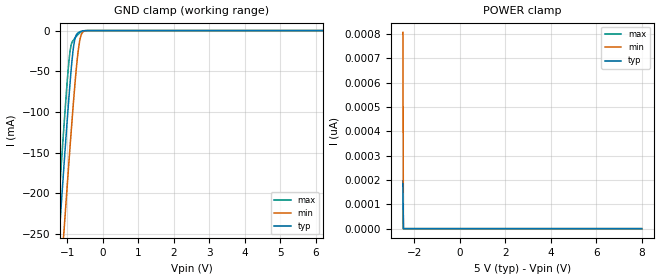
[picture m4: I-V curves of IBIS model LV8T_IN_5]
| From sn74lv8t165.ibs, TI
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[Model]   LV8T_IN_5
Model_type   Input
Vinl = 0.8
Vinh = 2
|   typ   min   max
C_comp   0.94pF   0.94pF   0.94pF
[Voltage Range]   5   4.5   5.5
[Temperature Range]   27   125   -40
[Power Clamp Reference]   5   4.5   5.5
[GND Clamp Reference]   0   0   0
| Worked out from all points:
|   GND clamp passes 1 mA (typ) near -0.62 V on its own axis
[GND Clamp]
|   Voltage   I(typ)   I(min)   I(max)
-2.5V     -1.102A    -1.155A    -1.067A
-1.292V   -294.1mA   -373.9mA   -246.2mA
-1.188V   -226.4mA   -306.9mA   -177.6mA
-1.083V   -160.1mA   -240.9mA   -111mA
-967mV    -90.42mA   -170.1mA   -44.5mA
-914.5mV  -60.98mA   -138.9mA   -23.57mA
-809.5mV  -15.97mA   -79.55mA   -10.72mA
-757mV    -6.46mA    -52.6mA    -7.795mA
-673mV    -2.071mA   -18.84mA   -3.804mA
-599.5mV  -718.5uA   -4.334mA   -1.428mA
-442mV    -12.39uA   -73.18uA   -11.72uA
8V        0A         0A         0A
[POWER Clamp]
|   Voltage   I(typ)   I(min)   I(max)
-2.5V     184.7pA    806.8pA    198pA
-2.479V   0A         0A         0A
-2.469V   0A         0A         0A
8V        0A         0A         0A
